
DATA_BLOCK DB3544
TITLE=
VERSION : 0.1

STRUCT
   CM_ID : STRING  [8 ] := '=VEN'; //COMPOSITE MACHINE
   STATION_ID : STRING  [8 ] := '++OP20'; //STATION - TRATTO - ZONE
   ELEMENT_ID : STRING  [8 ] := '+82CLT81'; //ELEMENT
   DB_ID : INT := 0 ; //DB SIZE OR TYPE
   PART_STYLE : STRING  [12 ]; //PART STYLE ON LAST STATION
   ACT_CYCLE_TIME : INT ; //ACTUAL CYCLE TIME FOR THIS STYLE
   COUNT_GOOD : INT ; //COUNTER GOOD PIECES
   COUNT_SCRAP : INT ; //COUNTER SCRAP PIECES
   SPARE_00 : ARRAY  [0 .. 15 ] OF //SPARE INTEGER
   INT ;
   SPARE_01 : ARRAY  [0 .. 17 ] OF //SPARE INTEGER
   INT ;
   CODE_EVENT : ARRAY  [0 .. 7 ] OF //CODE EVENT - EXTENDED FAULT CODE DIAGNOSTIC
   INT ;
   EVENT : STRUCT
      E0000 : BOOL ; //+82CLT81-B40N;MS.GENERALI ERRORE;1

E0001 : BOOL ; //+82CLT81-B40N;MS.GENERALI AVVERTIMENTO;2

E0002 : BOOL ; //+82CLT81-B40N; MS.  TEMPERATURA OK;58

E0003 : BOOL ; //+82CLT81-B40N; MS. MS_03;58

E0004 : BOOL ; //+82CLT81-B40N; MS. MS_04;58

E0005 : BOOL ; //+82CLT81-B40N; MS. MS_05;58

E0006 : BOOL ; //+82CLT81-B40N; MS. MS_06;58

E0007 : BOOL ; //+82CLT81-B40N; MS. MS_07;58

E0008 : BOOL ; //+82CLT81-B40N;MS.L03 MASSIMO AVVERTIMENTO;2

E0009 : BOOL ; //+82CLT81-B40N;MS.L02 MINIMO AVVERTIMENTO;2

E0010 : BOOL ; //+82CLT81-B40N; MS. MS_12;58

E0011 : BOOL ; //+82CLT81-B40N; MS. MS_13;58

E0012 : BOOL ; //+82CLT81-B40N; MS. MS_14;58

E0013 : BOOL ; //+82CLT81-B40N; MS. MS_15;58

E0014 : BOOL ; //+82CLT81-B40N; MS. MS_16;58

E0015 : BOOL ; //+82CLT81-B40N; MS. TEMPERATURA TROPPO ALTA;58

E0016 : BOOL ; //+82CLT81-B40N;ME.L04 MASSIMO ERRORE;1

E0017 : BOOL ; //+82CLT81-B40N;ME.L01 MINIMO ERRORE;1

E0018 : BOOL ; //+82CLT81-B40N; ME. ME_02;58

E0019 : BOOL ; //+82CLT81-B40N; ME. ME_03;58

E0020 : BOOL ; //+82CLT81-B40N; ME. ME_04;58

E0021 : BOOL ; //+82CLT81-B40N; ME. ME_05;58

E0022 : BOOL ; //+82CLT81-B40N; ME. ME_06;58

E0023 : BOOL ; //+82CLT81-B40N; ME. ME_07;58

E0024 : BOOL ; //+82CLT81-B40N; ME. ME_10;58

E0025 : BOOL ; //+82CLT81-B40N; ME. ME_11;58

E0026 : BOOL ; //+82CLT81-B40N; ME. ME_12;58

E0027 : BOOL ; //+82CLT81-B40N; ME. ME_13;58

E0028 : BOOL ; //+82CLT81-B40N; ME. ME_14;58

E0029 : BOOL ; //+82CLT81-B40N; ME. ME_15;58

E0030 : BOOL ; //+82CLT81-B40N; ME. ME_16;58

E0031 : BOOL ; //+82CLT81-B40N; ME. ME_17;58
E0032 : BOOL ;
E0033 : BOOL ;
E0034 : BOOL ;
E0035 : BOOL ;
E0036 : BOOL ;
E0037 : BOOL ;
E0038 : BOOL ;
E0039 : BOOL ;
E0040 : BOOL ;
E0041 : BOOL ;
E0042 : BOOL ;
E0043 : BOOL ;
E0044 : BOOL ;
E0045 : BOOL ;
E0046 : BOOL ;
E0047 : BOOL ;
E0048 : BOOL ;
E0049 : BOOL ;
E0050 : BOOL ;
E0051 : BOOL ;
E0052 : BOOL ;
E0053 : BOOL ;
E0054 : BOOL ;
E0055 : BOOL ;
E0056 : BOOL ;
E0057 : BOOL ;
E0058 : BOOL ;
E0059 : BOOL ;
E0060 : BOOL ;
E0061 : BOOL ;
E0062 : BOOL ;
E0063 : BOOL ;
END_STRUCT;
END_STRUCT;
BEGIN
CM_ID := '=VEN';
STATION_ID := '++OP20';
ELEMENT_ID := '+82CLT81';
DB_ID := 0 ;
PART_STYLE := '';
ACT_CYCLE_TIME := 0;
COUNT_GOOD := 0;
COUNT_SCRAP := 0;
SPARE_00[0] := 0;
SPARE_00[1] := 0;
SPARE_00[2] := 0;
SPARE_00[3] := 0;
SPARE_00[4] := 0;
SPARE_00[5] := 0;
SPARE_00[6] := 0;
SPARE_00[7] := 0;
SPARE_00[8] := 0;
SPARE_00[9] := 0;
SPARE_00[10] := 0;
SPARE_00[11] := 0;
SPARE_00[12] := 0;
SPARE_00[13] := 0;
SPARE_00[14] := 0;
SPARE_00[15] := 0;
SPARE_01[0] := 0;
SPARE_01[1] := 0;
SPARE_01[2] := 0;
SPARE_01[3] := 0;
SPARE_01[4] := 0;
SPARE_01[5] := 0;
SPARE_01[6] := 0;
SPARE_01[7] := 0;
SPARE_01[8] := 0;
SPARE_01[9] := 0;
SPARE_01[10] := 0;
SPARE_01[11] := 0;
SPARE_01[12] := 0;
SPARE_01[13] := 0;
SPARE_01[14] := 0;
SPARE_01[15] := 0;
SPARE_01[16] := 0;
SPARE_01[17] := 0;
CODE_EVENT[0] := 0;
CODE_EVENT[1] := 0;
CODE_EVENT[2] := 0;
CODE_EVENT[3] := 0;
CODE_EVENT[4] := 0;
CODE_EVENT[5] := 0;
CODE_EVENT[6] := 0;
CODE_EVENT[7] := 0;
EVENT.E0000 := FALSE;
EVENT.E0001 := FALSE;
EVENT.E0002 := FALSE;
EVENT.E0003 := FALSE;
EVENT.E0004 := FALSE;
EVENT.E0005 := FALSE;
EVENT.E0006 := FALSE;
EVENT.E0007 := FALSE;
EVENT.E0008 := FALSE;
EVENT.E0009 := FALSE;
EVENT.E0010 := FALSE;
EVENT.E0011 := FALSE;
EVENT.E0012 := FALSE;
EVENT.E0013 := FALSE;
EVENT.E0014 := FALSE;
EVENT.E0015 := FALSE;
EVENT.E0016 := FALSE;
EVENT.E0017 := FALSE;
EVENT.E0018 := FALSE;
EVENT.E0019 := FALSE;
EVENT.E0020 := FALSE;
EVENT.E0021 := FALSE;
EVENT.E0022 := FALSE;
EVENT.E0023 := FALSE;
EVENT.E0024 := FALSE;
EVENT.E0025 := FALSE;
EVENT.E0026 := FALSE;
EVENT.E0027 := FALSE;
EVENT.E0028 := FALSE;
EVENT.E0029 := FALSE;
EVENT.E0030 := FALSE;
EVENT.E0031 := FALSE;
EVENT.E0032 := FALSE;
EVENT.E0033 := FALSE;
EVENT.E0034 := FALSE;
EVENT.E0035 := FALSE;
EVENT.E0036 := FALSE;
EVENT.E0037 := FALSE;
EVENT.E0038 := FALSE;
EVENT.E0039 := FALSE;
EVENT.E0040 := FALSE;
EVENT.E0041 := FALSE;
EVENT.E0042 := FALSE;
EVENT.E0043 := FALSE;
EVENT.E0044 := FALSE;
EVENT.E0045 := FALSE;
EVENT.E0046 := FALSE;
EVENT.E0047 := FALSE;
EVENT.E0048 := FALSE;
EVENT.E0049 := FALSE;
EVENT.E0050 := FALSE;
EVENT.E0051 := FALSE;
EVENT.E0052 := FALSE;
EVENT.E0053 := FALSE;
EVENT.E0054 := FALSE;
EVENT.E0055 := FALSE;
EVENT.E0056 := FALSE;
EVENT.E0057 := FALSE;
EVENT.E0058 := FALSE;
EVENT.E0059 := FALSE;
EVENT.E0060 := FALSE;
EVENT.E0061 := FALSE;
EVENT.E0062 := FALSE;
EVENT.E0063 := FALSE;
END_DATA_BLOCK
